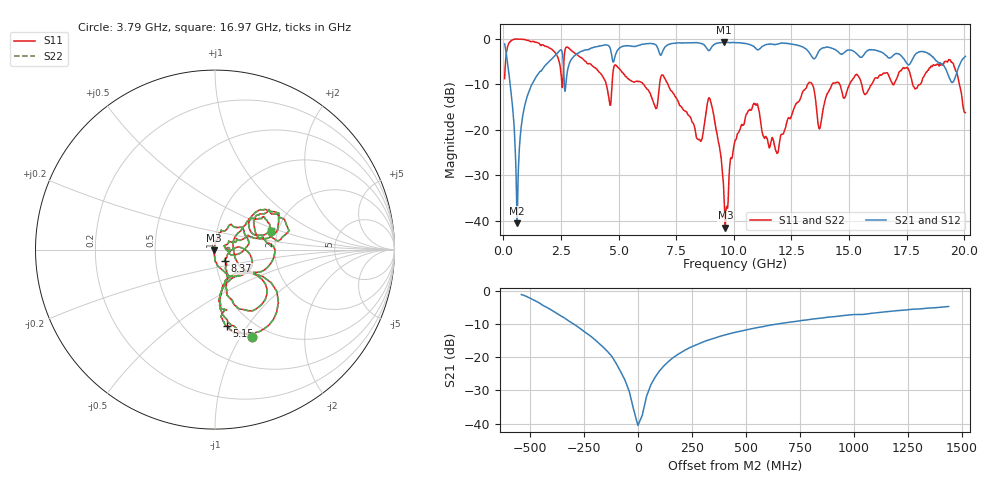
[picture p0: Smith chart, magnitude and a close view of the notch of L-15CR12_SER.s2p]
! P/N: L-15CR12JE
! Measured by Marlon
! Oct. 14, 2003
! Measure with Series-through-Fixture
#	mhz	s	ma	r	50
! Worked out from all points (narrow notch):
!   1001 points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, 50 MHz to 20.05 GHz, reference 50 ohm
!   highest |S21| = -0.69 dB at 9.57 GHz (marker M1); lowest = -40.6 dB at 590 MHz (marker M2)
!   notch at M2: 38.2 dB deep, 243 MHz wide at half that depth
!   lowest |S11| = -41.6 dB at 9.63 GHz (marker M3), VSWR 1.02, Z = 49.2 - j0.347 ohm
!   |S11| at or under -10 dB: 6.091 GHz to 6.775 GHz (684.3 MHz wide, 10.6 % of centre); 7.141 GHz to 13.2 GHz (6.062 GHz wide, 59.6 % of centre); 13.41 GHz to 14.26 GHz (855.3 MHz wide, 6.18 % of centre)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
!   |S22| runs from -41.6 to 0.0 dB; largest |S21 - S12| = 0
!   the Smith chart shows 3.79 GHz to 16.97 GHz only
!   S11 on the Smith chart (normalised r, x): 3.79 GHz: 0.82, -1.12; 5.15 GHz: 0.78, -0.81; 8.37 GHz: 1.11, -0.14; 16.97 GHz: 1.83, +0.42
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50  0.3668 64.3  0.8835 -20.3  0.8835 -20.3  0.3668 64.3
590  1 1.1  0.00937 0.0  0.00937 0.0  1 1.1
1290  0.9421 -21.2  0.3372 63.9  0.3372 63.9  0.9421 -21.2
3390  0.6218 -59.2  0.7322 31.3  0.7322 31.3  0.6218 -59.2
3790  0.5297 -67.3  0.793 24.4  0.793 24.4  0.5297 -67.3
4590  0.2114 -76.4  0.8318 2.4  0.8318 2.4  0.2114 -76.4
5150  0.4299 -81.0  0.8265 14.3  0.8265 14.3  0.4299 -81.0
6730  0.246 -32.4  0.7514 -11.5  0.7514 -11.5  0.246 -32.4
8370  0.08345 -48.3  0.9146 -13.5  0.9146 -13.5  0.08345 -48.3
8990  0.2075 -43.3  0.7825 -10.7  0.7825 -10.7  0.2075 -43.3
9570  0.01872 -106.8  0.9237 -17.5  0.9237 -17.5  0.01872 -106.8
9630  0.00835 -155.1  0.9204 -18.5  0.9204 -18.5  0.00835 -155.1
10050  0.0756 78.3  0.9111 -22.3  0.9111 -22.3  0.0756 78.3
10930  0.1937 33.4  0.8021 -30.3  0.8021 -30.3  0.1937 33.4
11870  0.05502 18.8  0.8768 -29.7  0.8768 -29.7  0.05502 18.8
13390  0.3209 -13.3  0.6408 -46.3  0.6408 -46.3  0.3209 -13.3
13730  0.1034 13.4  0.7601 -32.9  0.7601 -32.9  0.1034 13.4
14330  0.3274 33.8  0.7757 -46.9  0.7757 -46.9  0.3274 33.8
16730  0.3902 11.3  0.6219 -53.4  0.6219 -53.4  0.3902 11.3
16970  0.3262 18.4  0.6784 -49.0  0.6784 -49.0  0.3262 18.4
19410  0.5761 -18.1  0.3478 -61.9  0.3478 -61.9  0.5761 -18.1
20050  0.1546 -17.0  0.6448 -45.5  0.6448 -45.5  0.1546 -17.0
